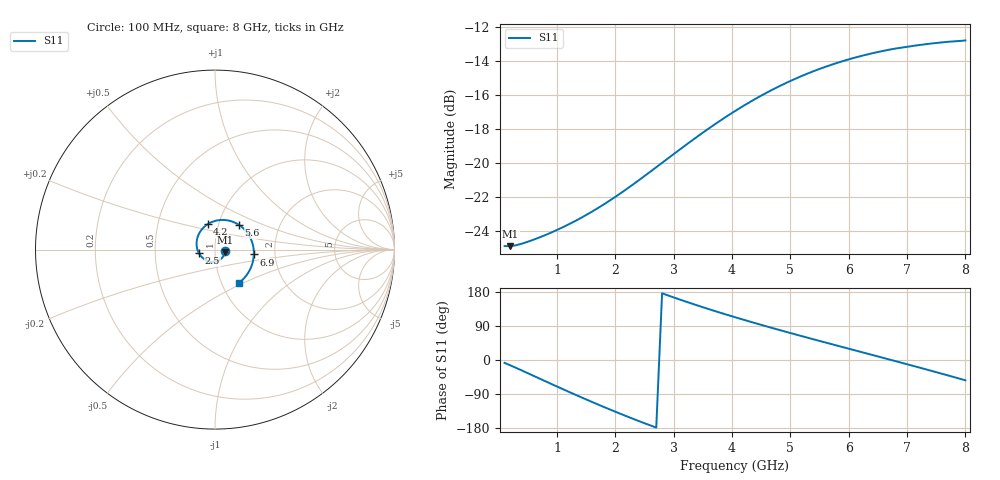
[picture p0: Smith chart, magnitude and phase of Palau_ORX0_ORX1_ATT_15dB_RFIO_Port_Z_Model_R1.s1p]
! Created Fri Oct  9 14:28:34 2020
! Palau ORX0/ORX1 RFIO Port Impedance Model.
! Attenuation  : 15 dB.
! Revision		: R1.
! Impedance Mode 	: Balanced Differential-Mode.
! Impedance Format 	: Series Equivalent Differential Impedance (SEDZ).
# hz S ma R 100
! 1 Port Network Data from SP1.SP block
! freq  magS11  angS11
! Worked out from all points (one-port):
!   80 points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, 100 MHz to 8 GHz, reference 100 ohm
!   lowest |S11| = -24.9 dB at 200 MHz (marker M1), VSWR 1.12, Z = 112 - j3.13 ohm
!   |S11| at or under -10 dB: start of sweep to end of sweep
!   S11 on the Smith chart (normalised r, x): 100 MHz: 1.12, -0.02; 2.5 GHz: 0.84, -0.03; 4.2 GHz: 0.89, +0.26; 5.6 GHz: 1.25, +0.36; 6.9 GHz: 1.55, -0.09; 8 GHz: 1.21, -0.47
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1e8  0.0569 -7.6
2e8  0.05687 -14.2
6e8  0.05946 -42.0
1.1e9  0.06468 -77.0
1.4e9  0.06872 -97.5
1.6e9  0.07188 -110.8
1.8e9  0.07545 -123.8
2.1e9  0.08163 -142.8
2.5e9  0.09147 -166.9
2.8e9  0.09997 176.0
3.1e9  0.1093 159.7
3.3e9  0.1159 149.3
3.6e9  0.1261 134.3
4.1e9  0.1437 110.6
4.2e9  0.1472 106.1
4.5e9  0.1576 92.7
4.7e9  0.1643 84.0
5.1e9  0.1771 67.0
5.3e9  0.1831 58.6
5.6e9  0.1915 46.2
5.8e9  0.1966 38.0
6.1e9  0.2037 25.7
6.5e9  0.2117 9.4
6.9e9  0.218 -7.1
7.1e9  0.2206 -15.3
7.5e9  0.225 -32.1
7.7e9  0.2268 -40.6
8e9  0.2289 -53.6
